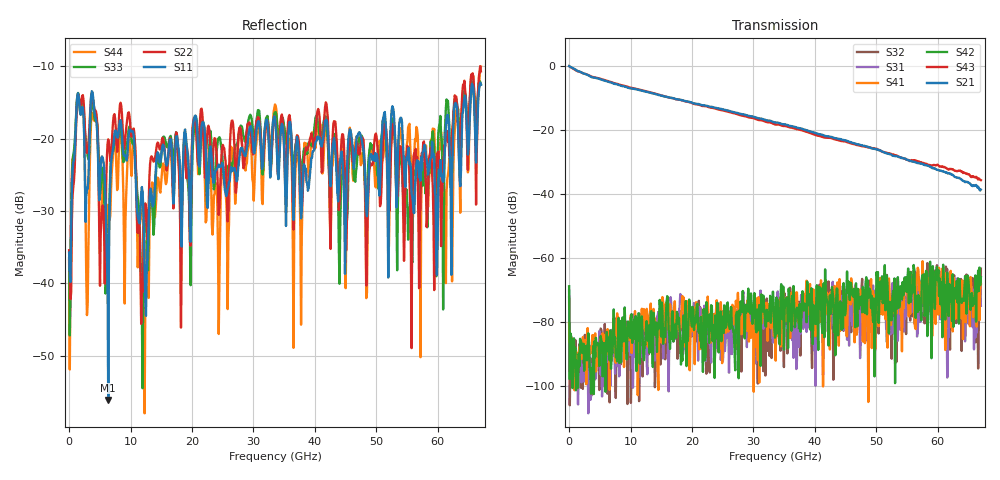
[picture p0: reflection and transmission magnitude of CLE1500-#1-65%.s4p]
!Keysight Technologies,N5247B,US50470101,A.16.20.02
!Date: Thursday, March 13, 2025 10:26:36
!Correction: S11(C  4-Port  )
!S12(C  4-Port  )
!S13(C  4-Port  )
!S14(C  4-Port  )
!S21(C  4-Port  )
!S22(C  4-Port  )
!S23(C  4-Port  )
!S24(C  4-Port  )
!S31(C  4-Port  )
!S32(C  4-Port  )
!S33(C  4-Port  )
!S34(C  4-Port  )
!S41(C  4-Port  )
!S42(C  4-Port  )
!S43(C  4-Port  )
!S44(C  4-Port  )
!S4P File: Measurements: <S11,S12,S13,S14>,
!<S21,S22,S23,S24>,
!<S31,S32,S33,S34>,
!<S41,S42,S43,S44>:
# Hz S  dB  R 50
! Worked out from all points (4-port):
!   601 points, 10 MHz to 67 GHz, reference 50 ohm
!   strongest paths, dB at 10 MHz, 16.76 GHz, 33.51 GHz, 50.25 GHz, 67 GHz:
!     S21: 0.0, -9.9, -17.6, -26.1, -38.6
!     S43: 0.0, -10.0, -18.2, -26.1, -35.6
!     S42: -68.8, -76.6, -84.8, -64.3, -65.9
!     S41: -80.2, -77.3, -77.5, -71.5, -67.9
!     S31: -70.1, -79.9, -80.5, -72.8, -74.9
!     S32: -72.1, -83.7, -84.9, -76.9, -63.3
!   lowest |S11| = -56.1 dB at 6.374 GHz (marker M1), VSWR 1.00, Z = 50 - j0.152 ohm
!   |S11| at or under -10 dB: start of sweep to end of sweep
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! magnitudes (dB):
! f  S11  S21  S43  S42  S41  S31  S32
! 10 MHz  -35.8  0.0  0.0  -68.8  -80.2  -70.1  -72.1
! 1.461 GHz  -13.7  -1.5  -1.6  -100.5  -89.5  -105.7  -94.9
! 6.374 GHz  -56.1  -4.9  -4.7  -84.8  -89.4  -92.5  -90.6
! 8.272 GHz  -17.5  -6.1  -5.8  -79.6  -83.7  -86.9  -83.8
! 11.84 GHz  -26.7  -7.7  -7.5  -78.2  -75.8  -90.8  -82.7
! 55.72 GHz  -27.6  -29.7  -29.3  -70.0  -69.7  -76.9  -72.2
! 67 GHz  -12.6  -38.6  -35.6  -65.9  -67.9  -74.9  -63.3
